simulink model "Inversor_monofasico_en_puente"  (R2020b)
settings: Solver=FixedStepAuto  StartTime=0.0  StopTime=0.033  FixedStep=0.0001  RelTol=1e-3
libraries: powerlib x10

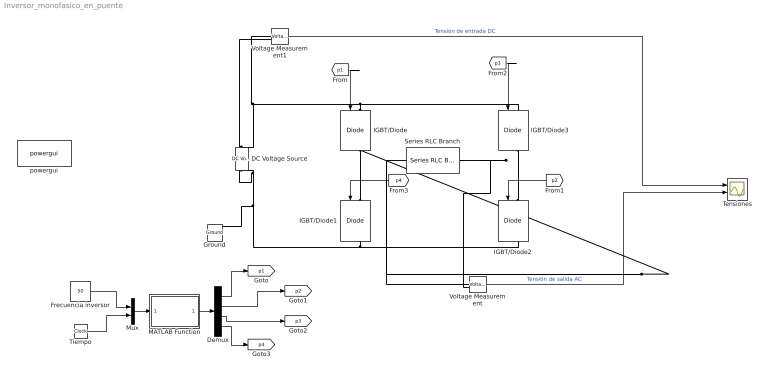
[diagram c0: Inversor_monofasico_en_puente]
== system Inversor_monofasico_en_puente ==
  DC Voltage Source : powerlib/Electrical Sources/DC Voltage Source  Amplitude=36  Measurements=Voltage
  Demux : Demux
  Frecuencia inversor : Constant  Value=50
  Ground : powerlib/Elements/Ground  LConnTagsString=a
  IGBT/Diode{,1..3} (4 alike) : powerlib/Power Electronics/IGBT//Diode  Ron=1e-3  Rs=1e5  Cs=inf  Measurements=on
  MATLAB Function : MATLAB Function  TreatAsAtomicUnit=on
  Mux : Mux  Inputs=2
  Series RLC Branch : powerlib/Elements/Series RLC Branch  LConnTagsString=__new0  RConnTagsString=__new0  BranchType=RL  Resistance=10  Inductance=0.025  SetiL0=off  InitialCurrent=0  Capacitance=1e-6  Setx0=off  InitialVoltage=0  Measurements=None
  Tensiones : Scope  NumInputPorts=2
  Tiempo : Clock
  Voltage Measurement : powerlib/Measurements/Voltage Measurement  PhasorSimulation=off  OutputType=Complex  PSBequivalent=0
  Voltage Measurement1 : powerlib/Measurements/Voltage Measurement  PhasorSimulation=off  OutputType=Complex  PSBequivalent=0
  powergui : powerlib/powergui  Priority=1  SimulationMode=Continuous  SampleTime=50e-6  frequency=60  Iterations=50  frequencyindice=0  Pbase=100e6  ErrMax=1e-4  UnitsV=kV  UnitsW=MW  buscounter=0  FunctionMessages=off  echomessages=off  EnableUseOfTLC=off  CurrentSourceSwitches=off  DisableSnubberDevices=off  DisableRonSwitches=off  DisableVfSwitches=off  DisplayEquations=off  AutomaticDiscreteSolvers=off  SolverType=Tustin/Backward Euler (TBE)  Interpol=off  ExternalGateDelay=off  methode=off  Ts=100  x0status=blocks  SPID=on  SwTol=0  HookPort=off  NonlinearTolerance=1e-4  nMaxIteration=100  ContinueOnMaxIteration=off  RestoreLinks=warning  ResistiveCurrentMeasurement=off  Frange=[0:2:500]  Ylog=off  Xlog=on  ShowGrid=off  save=off  variable=ZData  structure=0  ZoomFFT=off  StartTime=0.0  cycles=1  DisplayStyle=1  fundamental=60  FreqAxis=off  MaxFrequency=1000  frequencyindicesteady=1  RmsSteady=1  display=off
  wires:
  [p1] -> IGBT/Diode/1
  [p3] -> IGBT/Diode3/1
  [p2] -> IGBT/Diode2/1
  [p4] -> IGBT/Diode1/1
  Mux/1 -> MATLAB Function/1(u)
  Frecuencia inversor/1 -> Mux/1
  Tiempo/1 -> Mux/2
  MATLAB Function/1(y) -> Demux/1
  Demux/1 -> [p1]
  Demux/4 -> [p4]
  Demux/3 -> [p3]
  Demux/2 -> [p2]
  Voltage Measurement/1 -> Tensiones/2  "Tensión de salida AC"
  Voltage Measurement1/1 -> Tensiones/1  "Tensión de entrada DC"
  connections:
  IGBT/Diode/RConn1 -- Voltage Measurement/LConn1 -- Series RLC Branch/LConn1 -- IGBT/Diode1/LConn1
  IGBT/Diode3/RConn1 -- Series RLC Branch/RConn1 -- Voltage Measurement/LConn2 -- IGBT/Diode2/LConn1
  IGBT/Diode/LConn1 -- IGBT/Diode3/LConn1 -- DC Voltage Source/RConn1 -- Voltage Measurement1/LConn1
  IGBT/Diode1/RConn1 -- IGBT/Diode2/RConn1 -- Ground/LConn1 -- Voltage Measurement1/LConn2 -- DC Voltage Source/LConn1

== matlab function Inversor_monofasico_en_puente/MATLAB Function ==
function y = fcn(u)
f=u(1);                 %frecuencia
w=2*pi*f;               %frecuencia angular
t=u(2);                 %Tiempo
angulo= w*t;            %Ángulo (rad)
CA=cos(angulo);         %coseno angulo
SA=sin(angulo);         %seno angulo

%Condiciones para que el ángulo varíe entre 0 y 2pi 
% en vez de crecer en rampa
if SA>0 && CA>=0
    ang=asind(SA);
elseif SA>0 && CA<=0
    ang=180-asind(SA);
elseif SA<0 && CA<=0
    ang=180-(asind(SA));
else
    ang=360+(asind(SA));
end

%Esquema de conmutación de interruptores
if(ang>0 && ang<=180)
    pulso1=1;
    pulso2=1;
    pulso3=0;
    pulso4=0;
else
    pulso1=0;
    pulso2=0;
    pulso3=1;
    pulso4=1;
end
y=[pulso1 pulso2 pulso3 pulso4];
